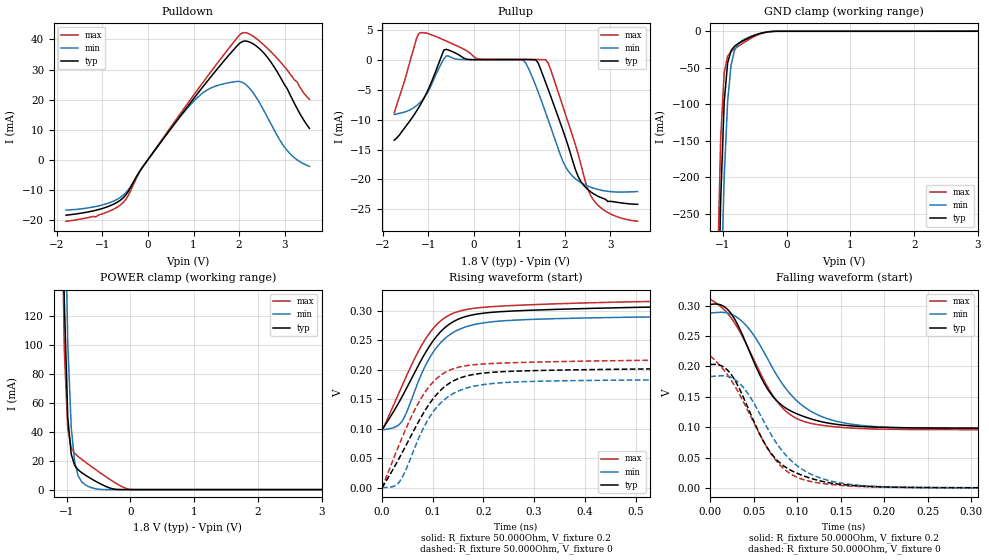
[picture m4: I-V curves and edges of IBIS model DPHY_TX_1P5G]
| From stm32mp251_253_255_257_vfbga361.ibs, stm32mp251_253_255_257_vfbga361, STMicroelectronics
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[Model] DPHY_TX_1P5G
Model_type   Output
Polarity   Non-Inverting
Enable   Active-High
C_comp 1.4pF   1.37pF   1.41pF
| This model is not intended for timing simulations.
| Warnings about Cref, Vref & Rref can be ignored
[Temperature Range]   25.000   -40.000   125.000
[Voltage Range]   1.800V   1.516V   2.030V
[GND Clamp Reference]   0.00V   0.00V   0.00V
[Pulldown Reference]   0.00V   0.00V   0.00V
[POWER Clamp Reference]   1.800V   1.516V   2.030V
[Pullup Reference]   1.800V   1.516V   2.030V
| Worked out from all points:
|   slope of the pulldown table from 0 to 0.27 V, typ, clamps not added: 48.6 ohm
|   slope of the pullup table from 0 to 0.27 V, typ, clamps not added: 40.7 kohm
|   GND clamp passes 1 mA (typ) near -0.31 V on its own axis
|   POWER clamp passes 1 mA (typ) near -0.31 V on its own axis
|   rising waveform, R_fixture 50.000Ohm, V_fixture 0.2: 20-80 % time 88.9ps typ, 71.9ps min, 82.8ps max; typ from 0.098 V to 0.31 V
|   rising waveform, R_fixture 50.000Ohm, V_fixture 0: 20-80 % time 84.7ps typ, 69.4ps min, 75.6ps max; typ from 0 V to 0.203 V
|   falling waveform, R_fixture 50.000Ohm, V_fixture 0.2: 20-80 % time 45.6ps typ, 55ps min, 49.1ps max; typ from 0.302 V to 0.098 V
|   falling waveform, R_fixture 50.000Ohm, V_fixture 0: 20-80 % time 46.7ps typ, 52.5ps min, 51ps max; typ from 0.203 V to 0 V
[GND Clamp]
-1.8V     -4.042A    -4.073A    -4.034A
-1.091V   -451.6mA   -607.8mA   -348.2mA
-1.036V   -231.6mA   -376.3mA   -146.6mA
-981.8mV  -97.78mA   -201.9mA   -57.02mA
-927.3mV  -43.35mA   -96.27mA   -34.12mA
-872.7mV  -26.43mA   -46.13mA   -27.69mA
-818.2mV  -20.42mA   -25.76mA   -23.97mA
-763.6mV  -17.02mA   -17.38mA   -20.69mA
-654.5mV  -11.72mA   -10.47mA   -14.49mA
-436.4mV  -3.482mA   -3.303mA   -4.29mA
-218.2mV  -146.9uA   -265.1uA   -132uA
3.545V    426.1nA    2.473uA    648.9uA
[Power Clamp]
-1.745V   4.178A     4.144A     4.305A
-1.091V   310.6mA    421.8mA    251.8mA
-1.036V   130.9mA    223.5mA    97.01mA
-981.8mV  50.29mA    102.3mA    42.42mA
-927.3mV  24.5mA     43.3mA     28.87mA
-872.7mV  16.75mA    18.99mA    25.02mA
-818.2mV  13.67mA    9.453mA    22.85mA
-709.1mV  10.1mA     3.359mA    19.17mA
-545.5mV  5.79mA     575.5uA    13.9mA
-327.3mV  1.19mA     3.793uA    7.229mA
-3uV      9.747nA    10.82nA    94.99uA
3.6V      -1.243uA   -14.78uA   -237.3nA
[Pulldown]
-1.8V     -18.49mA   -16.79mA   -20.54mA
-1.145V   -16.87mA   -15.61mA   -19.07mA
-545.5mV  -12.76mA   -11.88mA   -14.3mA
-163.6mV  -3.435mA   -3.542mA   -3.617mA
600mV     12.28mA    12.18mA    12.96mA
1.091V    22.02mA    20.73mA    23.3mA
1.527V    30.28mA    24.68mA    32.17mA
2.073V    39.32mA    25.73mA    42.18mA
2.291V    38.7mA     22.63mA    41.27mA
2.618V    34.15mA    14.25mA    37.13mA
3.055V    23.7mA     3.064mA    29.91mA
3.545V    10.4mA     -2.252mA   20.05mA
[Pullup]
-1.745V   -13.43mA   -9.108mA   -8.84mA
-1.2V     -7.861mA   -7.271mA   4.52mA
-654.5mV  1.717mA    221.3uA    3.412mA
109.1mV   108.7uA    79.91uA    207.6uA
1.091V    102.7uA    -16.32uA   159.1uA
1.364V    71.88uA    -4.288mA   132.1uA
1.582V    -3.769mA   -8.826mA   89.18uA
2.018V    -13.07mA   -17.9mA    -9.136mA
2.291V    -19.47mA   -20.24mA   -15.68mA
2.564V    -22.08mA   -21.32mA   -22.65mA
2.945V    -23.73mA   -22.02mA   -25.58mA
3.6V      -24.21mA   -22.07mA   -27.06mA
[Ramp]
R_load=50.000Ohm
dV/dt_r   123.703mV/64.000ps  113.576mV/81.000ps  130.819mV/52.000ps
dV/dt_f   122.219mV/51.000ps  112.106mV/62.000ps  129.869mV/47.000ps
[Rising waveform]
R_fixture=50.000Ohm
V_fixture=0.2
0s        98.31mV    98mV       95.86mV
26ps      133.6mV    102.7mV    146.2mV
40ps      154.9mV    113.4mV    173.5mV
66ps      197.9mV    167.5mV    221.6mV
88ps      232.2mV    210.9mV    255mV
118ps     266.3mV    247.8mV    284.2mV
156ps     287.4mV    269.6mV    299.8mV
212ps     296.7mV    280.5mV    306.3mV
318ps     301.3mV    285.7mV    310.7mV
1ns       310.1mV    291.9mV    319.4mV
[Rising waveform]
R_fixture=50.000Ohm
V_fixture=0
0s        -171.2uV   -57.09uV   -194uV
24ps      34.71mV    2.725mV    52.18mV
36ps      53.38mV    12.09mV    77.58mV
60ps      92.67mV    58.04mV    124.1mV
80ps      124mV      98.29mV    155.6mV
112ps     162mV      140.3mV    188mV
150ps     184.6mV    163.5mV    203.9mV
204ps     194.5mV    175.2mV    209.8mV
300ps     198.3mV    180.2mV    212.7mV
1ns       203mV      183.3mV    217.6mV
[Falling waveform]
R_fixture=50.000Ohm
V_fixture=0.2
0s        302.3mV    288.2mV    311mV
20ps      293.9mV    288mV      287.4mV
38ps      249.1mV    272.5mV    246.7mV
62ps      172.4mV    223.1mV    176.7mV
80ps      138.8mV    177.8mV    136.7mV
100ps     121.8mV    143mV      113.9mV
126ps     109.7mV    118.8mV    103.6mV
168ps     101.5mV    103.8mV    98.07mV
236ps     98.81mV    98.63mV    96.1mV
998ps     98.45mV    97.91mV    95.88mV
[Falling waveform]
R_fixture=50.000Ohm
V_fixture=0
0s        203.2mV    183.5mV    217.7mV
18ps      196.4mV    184.3mV    189.9mV
34ps      162.1mV    171.8mV    153.2mV
60ps      79.95mV    113.7mV    79.76mV
78ps      43.96mV    70.03mV    41.09mV
98ps      25.2mV     38.69mV    18.67mV
124ps     12.38mV    17.58mV    8.306mV
164ps     3.863mV    5.25mV     2.75mV
230ps     707.1uV    821.5uV    524.5uV
998ps     12.58uV    68.4uV     6.48uV
